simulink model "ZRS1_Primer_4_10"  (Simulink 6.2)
settings: Solver=ode45  StartTime=0.0  StopTime=10.0  FixedStep=1.e-5  MaxStep=0.01  RelTol=1.e-6
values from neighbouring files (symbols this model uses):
  kp = 19    [ZRS1_Primer4_9.m]    (also in ZRS1_Primer4_10_1.m = 18; ZRS1_Primer4_10_2.m = 18; ZRS1_Primer4_10_nih_preiz.m = 30)
  referenca = 0    [ZRS1_Primer4_9.m]    (also in ZRS1_Primer4_10_1.m = 1; ZRS1_Primer4_10_2.m = 1; ZRS1_Primer4_10_nih_preiz.m = 1)
  td = 4/19    (= 0.210526315789)    [ZRS1_Primer4_9.m]    (also in ZRS1_Primer4_10_1.m = 0.351; ZRS1_Primer4_10_2.m = 0.7692; ZRS1_Primer4_10_nih_preiz.m = 0)
  ti = 2    [ZRS1_Primer4_9.m]    (also in ZRS1_Primer4_10_1.m = 1.405; ZRS1_Primer4_10_2.m = 3.077; ZRS1_Primer4_10_nih_preiz.m = inf)

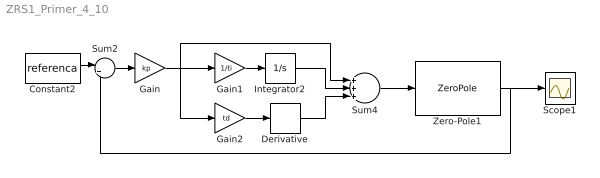
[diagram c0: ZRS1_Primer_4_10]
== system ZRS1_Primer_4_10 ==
  Constant2 : Constant  Value=referenca
  Derivative : Derivative
  Gain : Gain  Gain=kp
  Gain1 : Gain  Gain=1/ti
  Gain2 : Gain  Gain=td
  Integrator2 : Integrator
  Scope1 : Scope
  Sum2 : Sum  Inputs=|+-
  Sum4 : Sum  Inputs=+++
  Zero-Pole1 : ZeroPole  Zeros=[]  Poles="[0 -1  -5]"  Gain=1
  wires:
  Constant2/1 -> Sum2/1
  Sum2/1 -> Gain/1
  Zero-Pole1/1 -> Sum2/2, Scope1/1
  Gain/1 -> Gain1/1, Sum4/1, Gain2/1
  Gain1/1 -> Integrator2/1
  Integrator2/1 -> Sum4/2
  Gain2/1 -> Derivative/1
  Derivative/1 -> Sum4/3
  Sum4/1 -> Zero-Pole1/1
